// ------------------------------------------------------------------
// File           : C:\Users\acer\Documents\116.awl
//
// Source File    : C:\Users\acer\Documents\116.var
// Generation Date: 6/17/2019  Time: 2:24:51 PM
// ------------------------------------------------------------------

DATA_BLOCK DB  122
VERSION : 0.0


STRUCT

 C1_SGA_actToolBasePos4_2:
   STRUCT
   SYNTAX_ID : BYTE := B#16#82;
   bereich_u_einheit : BYTE := B#16#41;
   spalte : WORD := W#16#2;
   zeile : WORD := W#16#4;
   bausteintyp : BYTE := B#16#73;
   ZEILENANZAHL : BYTE := B#16#1;
   typ : BYTE := B#16#F;
   laenge : BYTE := B#16#8;
   END_STRUCT ;

 C1_SGA_actToolBasePos5_2:
   STRUCT
   SYNTAX_ID : BYTE := B#16#82;
   bereich_u_einheit : BYTE := B#16#41;
   spalte : WORD := W#16#2;
   zeile : WORD := W#16#5;
   bausteintyp : BYTE := B#16#73;
   ZEILENANZAHL : BYTE := B#16#1;
   typ : BYTE := B#16#F;
   laenge : BYTE := B#16#8;
   END_STRUCT ;

 END_STRUCT ;

BEGIN
END_DATA_BLOCK
